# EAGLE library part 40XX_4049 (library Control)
Hex inverting BUFFER
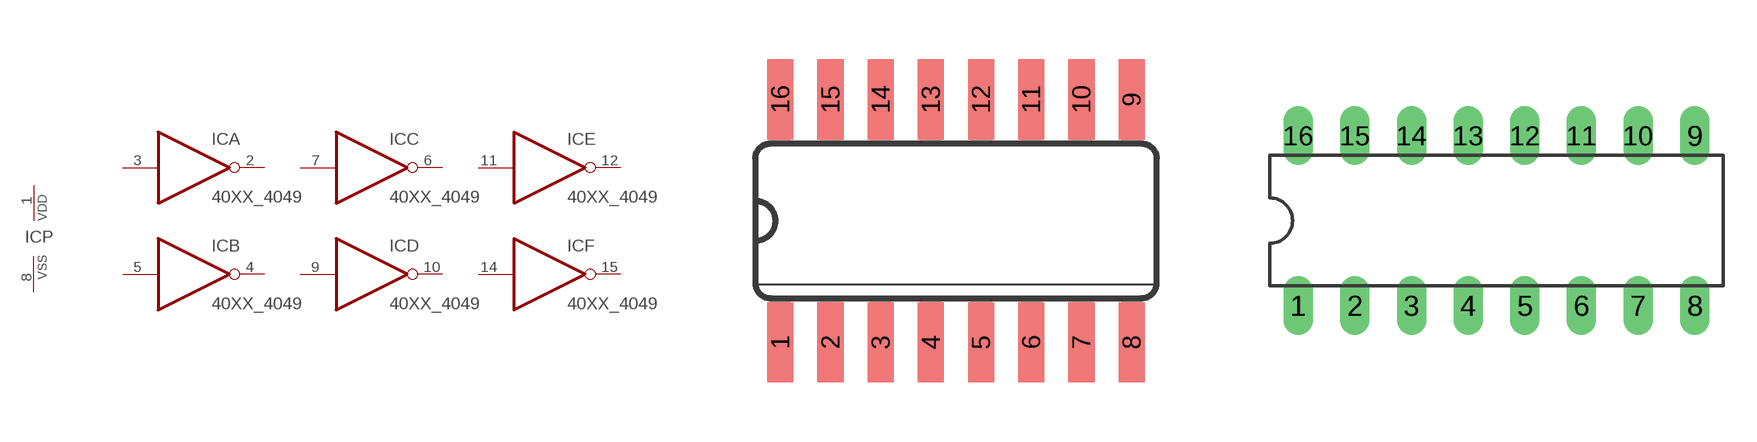
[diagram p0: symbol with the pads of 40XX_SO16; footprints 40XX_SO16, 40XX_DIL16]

Designator prefix IC; gates A=40XX_4049 B=40XX_4049 C=40XX_4049 D=40XX_4049 E=40XX_4049 F=40XX_4049 P=40XX_PWRN

## 40XX_4049D  [40XX_SO16]
1  P:VDD  pwr
2  A:O  out
3  A:I  in
4  B:O  out
5  B:I  in
6  C:O  out
7  C:I  in
8  P:VSS  pwr
9  D:I  in
10  D:O  out
11  E:I  in
12  E:O  out
14  F:I  in
15  F:O  out

## 40XX_4049N  [40XX_DIL16]
Pads as for 40XX_SO16

## Footprint 40XX_SO16 (pad centres in mm)
Small Outline package 150 mil
smd 0.66 x 2.032: 1 -4.445,-3.073; 2 -3.175,-3.073; 3 -1.905,-3.073; 4 -0.635,-3.073; 5 0.635,-3.073; 6 1.905,-3.073; 7 3.175,-3.073; 8 4.445,-3.073; 9 4.445,3.073; 10 3.175,3.073; 11 1.905,3.073; 12 0.635,3.073; 13 -0.635,3.073; 14 -1.905,3.073; 15 -3.175,3.073; 16 -4.445,3.073

## Footprint 40XX_DIL16 (pad centres in mm)
Dual In Line Package
drill 0.813 long: 1 -8.89,-3.81; 2 -6.35,-3.81; 3 -3.81,-3.81; 4 -1.27,-3.81; 5 1.27,-3.81; 6 3.81,-3.81; 7 6.35,-3.81; 8 8.89,-3.81; 9 8.89,3.81; 10 6.35,3.81; 11 3.81,3.81; 12 1.27,3.81; 13 -1.27,3.81; 14 -3.81,3.81; 15 -6.35,3.81; 16 -8.89,3.81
